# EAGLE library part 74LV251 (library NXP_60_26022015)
8-input multiplexer; 3-state The 74LV251 is a low-voltage Si-gate CMOS device and is pin and function compatible with 74HC/HCT251. The 74LV251 is an 8-input multiplexer with 8 binary inputs (I0 to I7), an output enable input (OE) and three select inputs (S0, S1, S2). One of the eight binary inputs is selected by the select inputs and is routed to the outputs (Y, Y). Both outputs are in the high impedance OFF-state (Z) when the output enable input is HIGH, allowing multiplexer expansion by tying the outputs. AAL Eindhoven MK
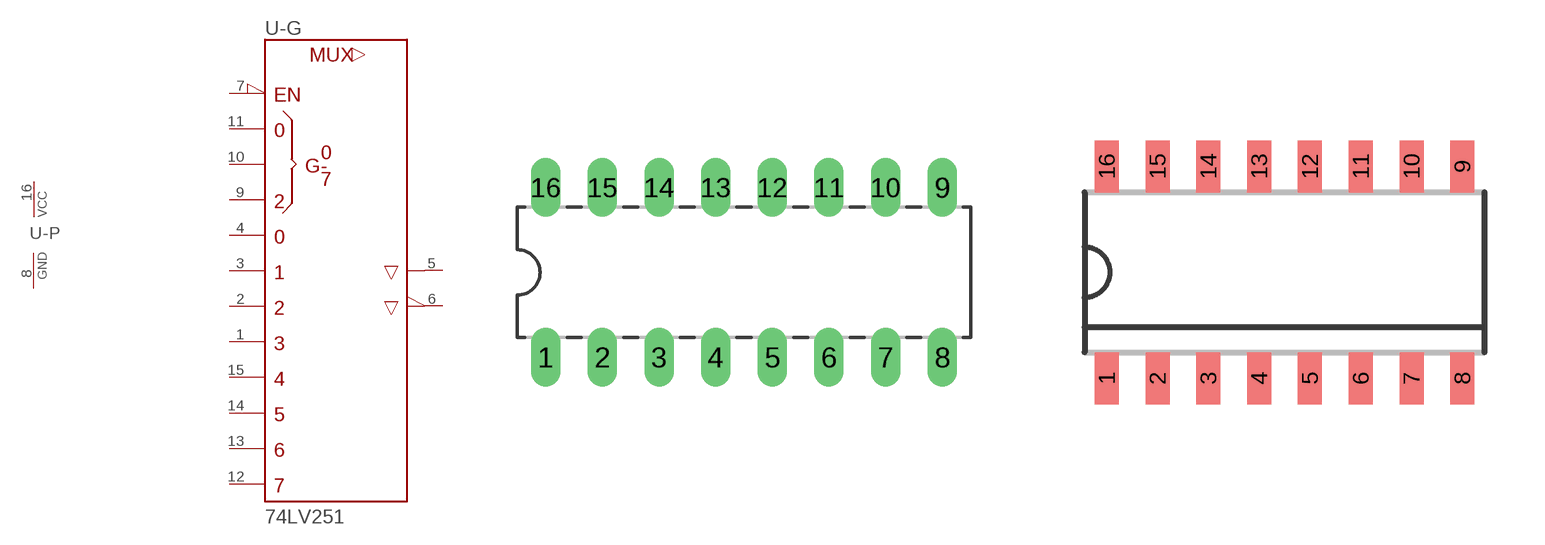
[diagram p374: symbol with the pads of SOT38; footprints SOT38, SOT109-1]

Designator prefix U; gates -G=251 -P=PWRN

## 74LV251N  [SOT38]
1  -G:D3  in
2  -G:D2  in
3  -G:D1  in
4  -G:D0  in
5  -G:Y  hiz
6  -G:W  hiz
7  -G:!G  in
8  -P:GND  pwr
9  -G:C  in
10  -G:B  in
11  -G:A  in
12  -G:D7  in
13  -G:D6  in
14  -G:D5  in
15  -G:D4  in
16  -P:VCC  pwr

## 74LV251D  [SOT109-1]
Pads as for SOT38

## 74LV251DP  [SOT338]
Pads as for SOT38

## 74LV251PW  [SOT403-1]
Pads as for SOT38

## Footprint SOT38 (pad centres in mm)
Dual In Line Package
drill 0.813 long: 1 -8.89,-3.81; 2 -6.35,-3.81; 3 -3.81,-3.81; 4 -1.27,-3.81; 5 1.27,-3.81; 6 3.81,-3.81; 7 6.35,-3.81; 8 8.89,-3.81; 9 8.89,3.81; 10 6.35,3.81; 11 3.81,3.81; 12 1.27,3.81; 13 -1.27,3.81; 14 -3.81,3.81; 15 -6.35,3.81; 16 -8.89,3.81

## Footprint SOT109-1 (pad centres in mm)
SOT109-1 SO16: plastic small outline package; 16 leads; body width 3.9 mm JEDEC: MS-012 IEC: 076E07
smd 0.6 x 1.3: 1 -4.445,-2.65; 2 -3.175,-2.65; 3 -1.905,-2.65; 4 -0.635,-2.65; 5 0.635,-2.65; 6 1.905,-2.65; 7 3.175,-2.65; 8 4.445,-2.65; 9 4.445,2.65; 10 3.175,2.65; 11 1.905,2.65; 12 0.635,2.65; 13 -0.635,2.65; 14 -1.905,2.65; 15 -3.175,2.65; 16 -4.445,2.65

## Footprint SOT338 (pad centres in mm)
SOT338 SSOP16: plastic shrink small outline package; 16 leads; body width 5.3 mm JEDEC: MO-150 IEC: --
smd 0.4 x 1.2: 1 -2.275,-3.45; 2 -1.625,-3.45; 3 -0.975,-3.45; 4 -0.325,-3.45; 5 0.325,-3.45; 6 0.975,-3.45; 7 1.625,-3.45; 8 2.275,-3.45; 9 2.275,3.45; 10 1.625,3.45; 11 0.975,3.45; 12 0.325,3.45; 13 -0.325,3.45; 14 -0.975,3.45; 15 -1.625,3.45; 16 -2.275,3.45

## Footprint SOT403-1 (pad centres in mm)
SOT403-1 TSSOP16: plastic thin shrink small outline package; 16 leads; body width 4.4 mm JEDEC: MO-153 IEC: ---
smd 0.6 x 1.35: 1 -2.375,-2.925; 8 2.375,-2.925; 9 2.375,2.925; 16 -2.375,2.925
smd 0.4 x 1.35: 2 -1.625,-2.925; 3 -0.975,-2.925; 4 -0.325,-2.925; 5 0.325,-2.925; 6 0.975,-2.925; 7 1.625,-2.925; 10 1.625,2.925; 11 0.975,2.925; 12 0.325,2.925; 13 -0.325,2.925; 14 -0.975,2.925; 15 -1.625,2.925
